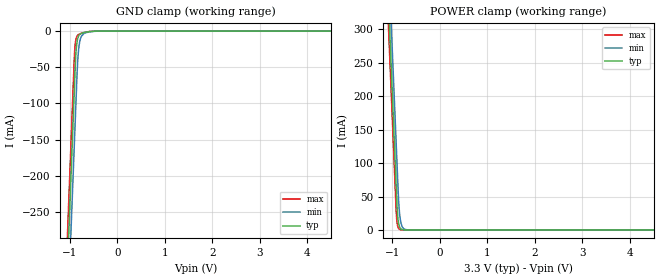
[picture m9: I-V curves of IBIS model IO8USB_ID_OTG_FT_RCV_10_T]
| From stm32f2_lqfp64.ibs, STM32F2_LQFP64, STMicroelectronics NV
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| *** New cell (Generated with 5.14beta1 (Sep 20 2010 13:23:23))
[Model]   IO8USB_ID_OTG_FT_RCV_10_T
Model_type Input
Polarity   Non-Inverting
Enable   Active-Low
| CAP_THRESHOLD on pad IOV33 is "CMOS" :
| Rising=10.0% of vddio   Falling=90.0% of vddio
| C_comp min and max val. don't necessarily correlate with the min and max pvt
| but are the smallest and greatest pad capacitance found.
| var   typ   min   max
C_comp   2.14545pF  2.04625pF  2.26745pF
Vinl = 800.0mV | Dummy value overriden by next lines
Vinh = 2.00V | Dummy value overriden by next lines
[Model Spec]
| TIME_THRESHOLD on pin ZIV12 is "CORE" :
| Rising=40.0% of vdd   Falling=60.0% of vdd
Vinl 1.48450V 1.23350V 1.61250V
Vinh 1.48450V 1.23350V 1.61250V
| variable   typ   min   max
[Temperature Range] 25.0 125.0 -40.0
| variable   typ   min   max
[Voltage Range] 3.3V 2.7V 3.6V
| variable   typ   min   max
[POWER Clamp Reference] 3.3V 2.7V 3.6V
| variable   typ   min   max
[GND Clamp Reference] 0V 0V 0V
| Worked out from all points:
|   GND clamp passes 1 mA (typ) near -0.62 V on its own axis
|   POWER clamp passes 1 mA (typ) near -0.81 V on its own axis
[POWER Clamp]
-3.3V     4.11A      4.173A     4.072A
-1.09V    352.5mA    415.9mA    314.5mA
-1.05V    284.5mA    347.9mA    246.5mA
-1.01V    216.5mA    279.9mA    178.5mA
-920mV    63.51mA    126.9mA    25.85mA
-900mV    31.51mA    92.9mA     9.552mA
-890mV    21.35mA    75.9mA     5.807mA
-870mV    9.804mA    44.01mA    2.146mA
-840mV    3.05mA     18.36mA    482.1uA
-780mV    295.2uA    3.194mA    24.34uA
-660mV    2.764uA    96.54uA    62.42nA
6.6V      0A         0A         0A
[GND Clamp]
-3.3V     -4.149A    -4.223A    -4.103A
-1.06V    -340.6mA   -415.4mA   -294.6mA
-940mV    -136.6mA   -211.4mA   -90.55mA
-900mV    -68.56mA   -143.4mA   -26.56mA
-880mV    -36.74mA   -109.4mA   -13.48mA
-870mV    -26.57mA   -92.41mA   -10.3mA
-840mV    -11.31mA   -44.9mA    -5.968mA
-820mV    -7.237mA   -26.99mA   -4.81mA
-790mV    -4.465mA   -13.32mA   -3.798mA
-700mV    -1.968mA   -2.918mA   -1.891mA
-350mV    -6.461uA   -36.64uA   -1.196uA
6.6V      9.456nA    1.186uA    63.86pA
